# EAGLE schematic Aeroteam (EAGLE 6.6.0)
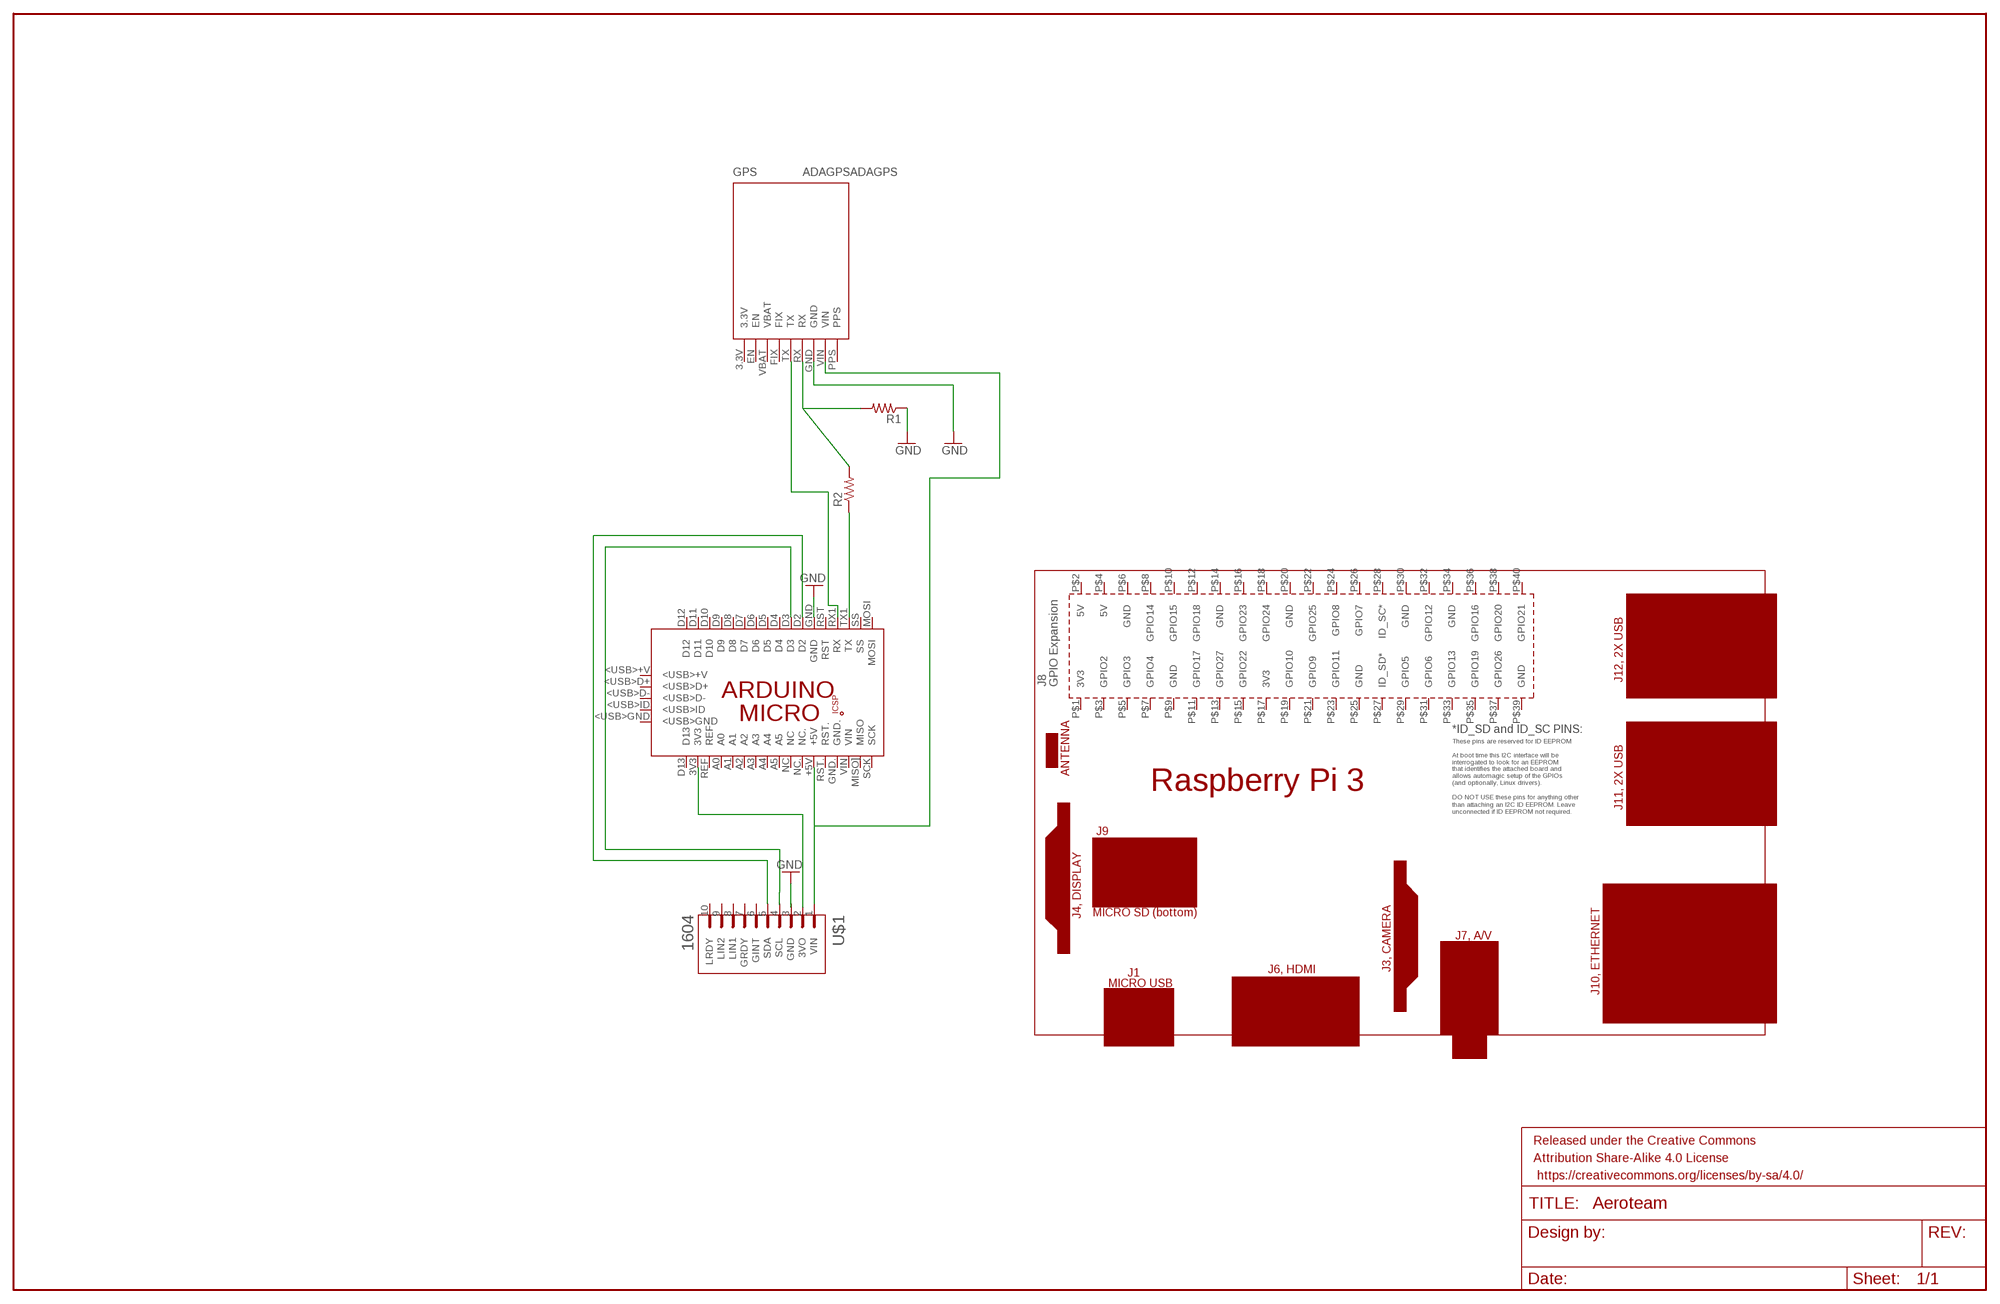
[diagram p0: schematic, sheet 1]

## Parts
FRAME1  FRAME-LEDGER  [CREATIVE_COMMONS]
GPS  ADAGPSADAGPS  [ADAGPS]
PCB1  ARDUINO_MICRO  [ARDUINO_MICRO]
PCB2  RPI3  [RPI3]
R1  RESISTORPTH-1/4W  [AXIAL-0.4]
R2  RESISTORPTH-1/4W  [AXIAL-0.4]
U$1  1604  [ADAFRUIT_1604]

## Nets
GND: GPS.GND PCB1.GND R1.P$1
N$1: PCB1.3V3
N$2: GPS.RX R1.P$2 R2.P$2
N$3: PCB1.TX1(TX) R2.P$1
N$4: PCB1.D3
N$5: GPS.VIN PCB1.+5V U$1.1(VIN)
N$6: GPS.TX PCB1.RX1(RX)
N$7: PCB1.D2 U$1.5(SDA)
Unconnected: GPS.3.3V GPS.EN GPS.FIX GPS.PPS GPS.VBAT PCB1.5V PCB1.<USB>+V PCB1.<USB>D+ PCB1.<USB>D- PCB1.<USB>GND PCB1.<USB>ID PCB1.A0 PCB1.A1 PCB1.A2 PCB1.A3 PCB1.A4 PCB1.A5 PCB1.D4 PCB1.D5 PCB1.D6 PCB1.D7 PCB1.D8 PCB1.D9 PCB1.D10 PCB1.D11 PCB1.D12 PCB1.D13 PCB1.GND. PCB1.GND_ PCB1.MISO. PCB1.MISO](MISO) PCB1.MOSI PCB1.MOSI. PCB1.NC PCB1.NC. PCB1.REF PCB1.RESET.. PCB1.RST PCB1.RST. PCB1.SCK PCB1.SCK. PCB1.SS PCB1.VIN PCB2.P$1(3V3) PCB2.P$2(5V) PCB2.P$3(GPIO2) PCB2.P$4(5V) PCB2.P$5(GPIO3) PCB2.P$6(GND) PCB2.P$7(GPIO4) PCB2.P$8(GPIO14) PCB2.P$9(GND) PCB2.P$10(GPIO15) PCB2.P$11(GPIO17) PCB2.P$12(GPIO18) PCB2.P$13(GPIO27) PCB2.P$14(GND) PCB2.P$15(GPIO22) PCB2.P$16(GPIO23) PCB2.P$17(3V3) PCB2.P$18(GPIO24) PCB2.P$19(GPIO10) PCB2.P$20(GND) PCB2.P$21(GPIO9) PCB2.P$22(GPIO25) PCB2.P$23(GPIO11) PCB2.P$24(GPIO8) PCB2.P$25(GND) PCB2.P$26(GPIO7) PCB2.P$27(ID_SD*) PCB2.P$28(ID_SC*) PCB2.P$29(GPIO5) PCB2.P$30(GND) PCB2.P$31(GPIO6) PCB2.P$32(GPIO12) PCB2.P$33(GPIO13) PCB2.P$34(GND) PCB2.P$35(GPIO19) PCB2.P$36(GPIO16) PCB2.P$37(GPIO26) PCB2.P$38(GPIO20) PCB2.P$39(GND) PCB2.P$40(GPIO21) U$1.4(SCL) U$1.6(GINT) U$1.7(GRDY) U$1.8(LIN1) U$1.9(LIN2) U$1.10(LRDY)

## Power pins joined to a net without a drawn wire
3VO: U$1.2(3VO)
GND: U$1.3(GND)

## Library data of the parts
FRAME1 = SparkFun-Aesthetics:FRAME-LEDGER: Schematic Frame
GPS = GPS:ADAGPS
PCB1 = E14_Arduino_revC:ARDUINO_MICRO: Device for representing an Arduino Micro board with a footprint in an EAGLE design. Created by Dave Young for Element14. More EAGLE documentation at: http://www.element14.com/community/community/knode/cadsoft_eagle
PCB2 = e14_Rpi3_RevA:RPI3: Device for Raspberry Pi 3 board created by Dave Young for www.element14.com More information and support community is available at https://www.element14.com/community/community/raspberry-pi
R1 R2 = SparkFun-Passives:RESISTOR: Resistor
U$1 = IMU:1604: Adafruit 10-DOF IMU Breakout - L3GD20H + LSM303 + BMP180; AVAILABILITY: Bad; DESCRIPTION: Adafruit 10-DOF IMU Breakout - L3GD20H + LSM303 + BMP180; MF: Adafruit Industries; MP: 1604; PACKAGE: None; PRICE: 26.66 USD

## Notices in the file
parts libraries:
SparkFun-Aesthetics: Licensing: Creative Commons ShareAlike 4.0 International - https://creativecommons.org/licenses/by-sa/4.0
SparkFun-Aesthetics: Released under the Creative Commons Attribution Share-Alike 4.0 License
SparkFun-Aesthetics: https://creativecommons.org/licenses/by-sa/4.0
